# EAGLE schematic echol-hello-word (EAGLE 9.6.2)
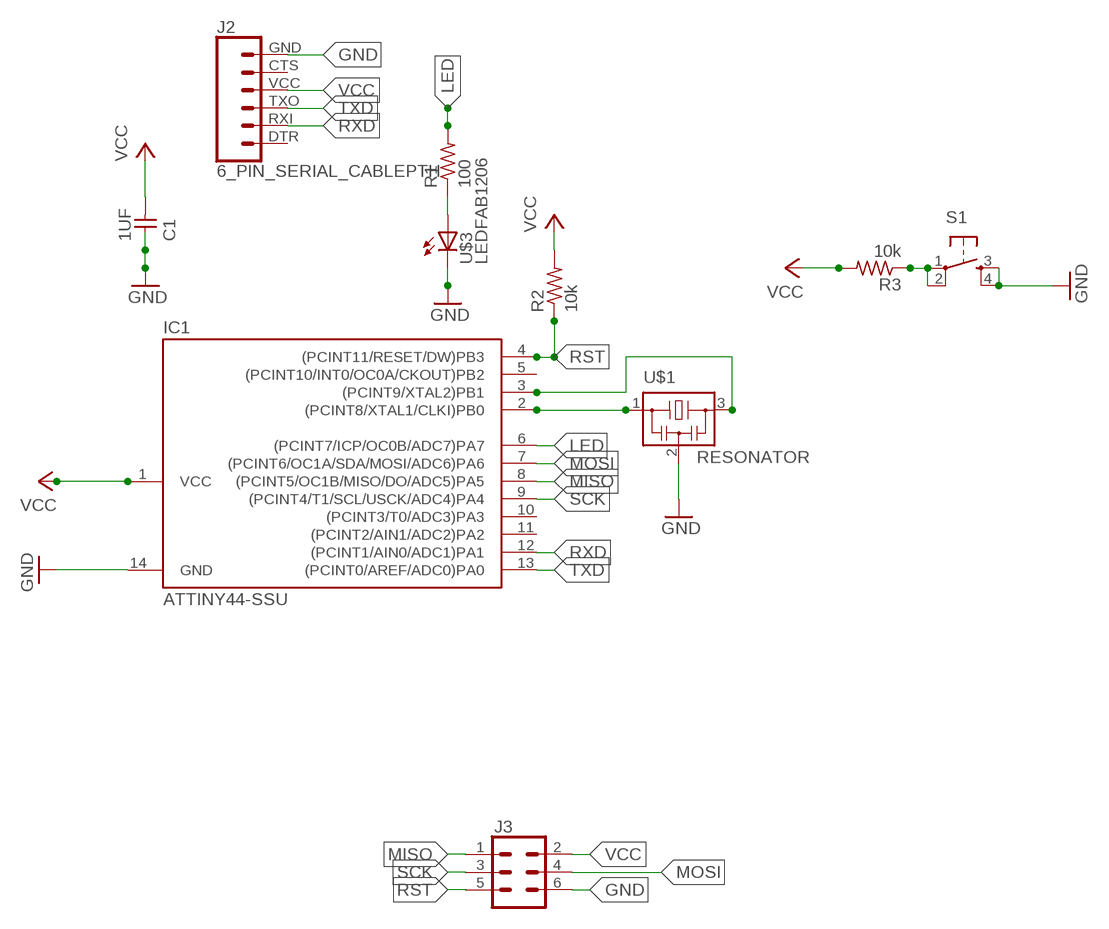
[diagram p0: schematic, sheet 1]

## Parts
C1  1UF  CAP-UNPOLARIZEDFAB  [C1206FAB]
IC1  ATTINY44-SSU  [SOIC14]
J2  6_PIN_SERIAL_CABLEPTH  [FTDI_BASIC]
J3  CONN_03X22X3_SILK_MALE_PTH  [2X3]
R1  100  RES-US1206FAB  [R1206FAB]
R2  10k  RES-US1206FAB  [R1206FAB]
R3  10k  RES-US1206FAB  [R1206FAB]
S1  6MM_SWITCH6MM_SWITCH  [6MM_SWITCH]
U$1  RESONATOR  [EFOBM]
U$3  LEDFAB1206  [LED1206FAB]

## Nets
GND: C1.1 IC1.14(GND) J2.GND J3.6 S1.3(S) S1.4(S1) U$1.2 U$3.2(C)
LED: IC1.6((PCINT7/ICP/OC0B/ADC7)PA7) R1.2
MISO: IC1.8((PCINT5/OC1B/MISO/DO/ADC5)PA5) J3.1
MOSI: IC1.7((PCINT6/OC1A/SDA/MOSI/ADC6)PA6) J3.4
N$1: R1.1 U$3.1(A)
N$2: IC1.2((PCINT8/XTAL1/CLKI)PB0) U$1.1
N$3: IC1.3((PCINT9/XTAL2)PB1) U$1.3
N$5: R3.1 S1.1(P) S1.2(P1)
RST: IC1.4((PCINT11/RESET/DW)PB3) J3.5 R2.1
RXD: IC1.12((PCINT1/AIN0/ADC1)PA1) J2.RXI
SCK: IC1.9((PCINT4/T1/SCL/USCK/ADC4)PA4) J3.3
TXD: IC1.13((PCINT0/AREF/ADC0)PA0) J2.TXO
VCC: C1.2 IC1.1(VCC) J2.VCC J3.2 R2.2 R3.2
Unconnected: IC1.5((PCINT10/INT0/OC0A/CKOUT)PB2) IC1.10((PCINT3/T0/ADC3)PA3) IC1.11((PCINT2/AIN1/ADC2)PA2) J2.CTS J2.DTR

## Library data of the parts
C1 = fab:CAP-UNPOLARIZED
IC1 = fab:ATTINY44
J2 = SparkFun-Connectors:6_PIN_SERIAL_CABLE: 6-pin header connection for use with the "FTDI BASIC" pinout - CABLE SIDE. Also known as "Arduino Serial Program Header". This is used on a design to provide a 6-pin connection point for serial communication usually from a USB cable (D+/D-) to these headers (RX/TX). It also has the remaining pins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
J3 = SparkFun-Connectors:CONN_03X2: Multi connection point. Often used as Generic Header-pin footprint for 0.1 inch spaced/style header connections You can populate with any combo of single row headers, but if you'd like an exact match, check these: Header - 2x3 (Male, 0.1") (PRT-12807) Header - 2x3 (Female, 0.1") (PRT-13010) 2x3 Pin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; PROD_ID: CONN-09701
R1-R3 = fab:RES-US: Resistor (US Symbol)
S1 = fab:6MM_SWITCH: OMRON SWITCH
U$1 = fab:RESONATOR
U$3 = fab:LED: LED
